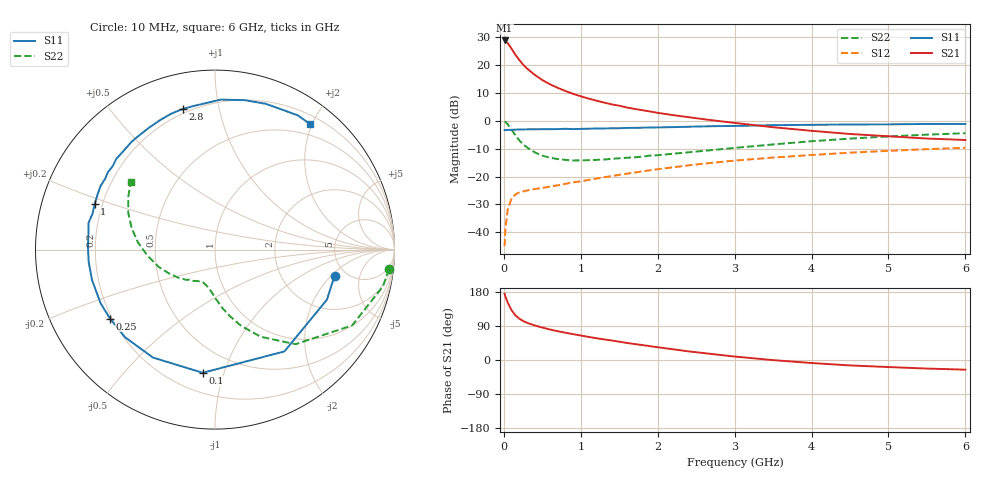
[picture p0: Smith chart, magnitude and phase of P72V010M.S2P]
! SIEMENS Small Signal Semiconductors
! BFP196
! Si NPN RF Bipolar Junction Transistor in SOT143
! VCE = 2 V  IC = 10 mA
! Common Emitter S-Parameters:  May  1996
# GHz  S  MA  R  50
!  f  S11  S21  S12  S22
! GHz  MAG  ANG  MAG  ANG  MAG  ANG  MAG  ANG
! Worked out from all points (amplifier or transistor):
!   36 points, 10 MHz to 6 GHz, reference 50 ohm
!   highest |S21| = 28.9 dB at 10 MHz (marker M1)
!   |S21| within 3 dB of that: start of sweep to 100.9 MHz
!   unconditionally stable (mu >= 1): 865.7 MHz to 3.409 GHz
!   at 250 MHz: K = 0.41, MSG = 22.8 dB, |S12| = -25.4 dB
!   at 1.4 GHz: K = 1.15, MAG = 10.6 dB, |S12| = -19.9 dB
!   at 6 GHz: K = 0.98, MSG = 1.4 dB, |S12| = -9.7 dB
!   S11 on the Smith chart (normalised r, x): 10 MHz: 4.02, -2.20; 100 MHz: 0.33, -0.85; 250 MHz: 0.19, -0.29; 1 GHz: 0.17, +0.18; 2.8 GHz: 0.18, +0.78; 6 GHz: 0.33, +1.98
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0.01  0.6819 -12.4  27.82 174.7  0.0056 85.3  0.9747 -6.4
0.02  0.6832 -24.1  27.12 167.6  0.0113 80.6  0.9583 -12.3
0.05  0.6866 -55.7  24.97 151.6  0.0255 65.2  0.8731 -28.9
0.1  0.6897 -95.7  19.79 131.4  0.0402 49.2  0.6922 -49.6
0.15  0.6937 -119.9  15.42 118.0  0.0477 40.3  0.5487 -62.3
0.2  0.6996 -135.7  12.47 109.3  0.0516 35.6  0.4489 -71.1
0.25  0.6998 -146.7  10.25 103.0  0.0539 33.1  0.3798 -77.4
0.3  0.7041 -154.8  8.737 98.3  0.056 32.3  0.3347 -82.1
0.4  0.7058 -166.1  6.732 91.3  0.0595 32.3  0.272 -89.5
0.5  0.7071 -174.3  5.412 85.6  0.0621 33.3  0.2365 -94.8
0.6  0.7079 178.9  4.538 80.5  0.0658 34.9  0.2177 -99.0
0.7  0.7102 173.2  3.919 75.9  0.0694 36.2  0.2059 -103.1
0.8  0.7205 168.1  3.439 72.0  0.0737 37.8  0.1993 -106.6
1  0.7171 159.2  2.761 64.6  0.0819 40.3  0.1948 -112.3
1.1  0.722 155.3  2.518 61.0  0.0868 41.3  0.1968 -115.2
1.6  0.747 137.3  1.736 45.0  0.1122 43.5  0.2172 -127.9
2.2  0.7713 119.0  1.266 28.3  0.1465 41.7  0.2567 -142.3
2.8  0.8043 102.8  0.989 13.6  0.1813 37.1  0.3071 -158.0
3.5  0.8362 87.8  0.768 -0.3  0.2189 29.7  0.3766 -174.7
4.5  0.8601 70.8  0.581 -14.3  0.2679 18.7  0.4795 165.5
5.5  0.8791 58.2  0.481 -22.6  0.3097 7.4  0.5649 148.9
6  0.8771 52.7  0.453 -25.5  0.3289 1.2  0.6007 141.4
